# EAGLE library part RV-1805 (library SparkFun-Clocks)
Micro Crystal Switzerland - RV-1805-C3 - Extremely low power RTC module This RTC IC has been specially designed for ultimate low current consumption of typically 60 nA @ VDD 3.0V for 32.768 kHz XTAL mode. Additionally, there is an RC-Mode consuming only 17nA and an autocalibrated RC-mode consuming 22nA which permits to operate this RTC module several hours at Backup Supply Voltage using low-cost MLCC. The very small SMT ceramic-package combines the 32.768 kHz crystal unit with the CMOS-based oscillator and real-time-clock IC.
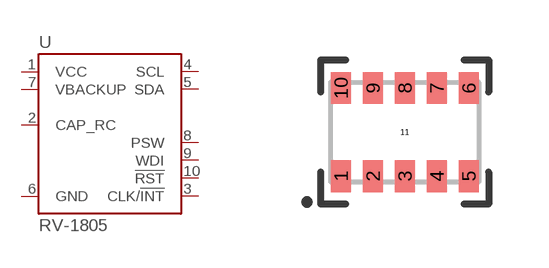
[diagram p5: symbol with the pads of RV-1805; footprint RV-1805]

Designator prefix U

## RV-1805 (PROD_ID: IC-13900)  [RV-1805]
1  VCC
2  CAP_RC
3  CLK/!INT
4  SCL
5  SDA
6  GND
7  VBACKUP
8  PSW
9  WDI
10  !RST

## Footprint RV-1805 (pad centres in mm)
SON 10-pin - Miniature SMT ceramic package Specifications: Pin count: [10] Pin pitch: [0.8mm] Area: [3.7mm x 2.5mm] Datasheet referenced for footprint
smd 0.5 x 0.8: 1 -1.6,-1.1; 2 -0.8,-1.1; 3 0,-1.1; 4 0.8,-1.1; 5 1.6,-1.1; 6 1.6,1.1; 7 0.8,1.1; 8 0,1.1; 9 -0.8,1.1; 10 -1.6,1.1
smd 0 x 0: 11 0,0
